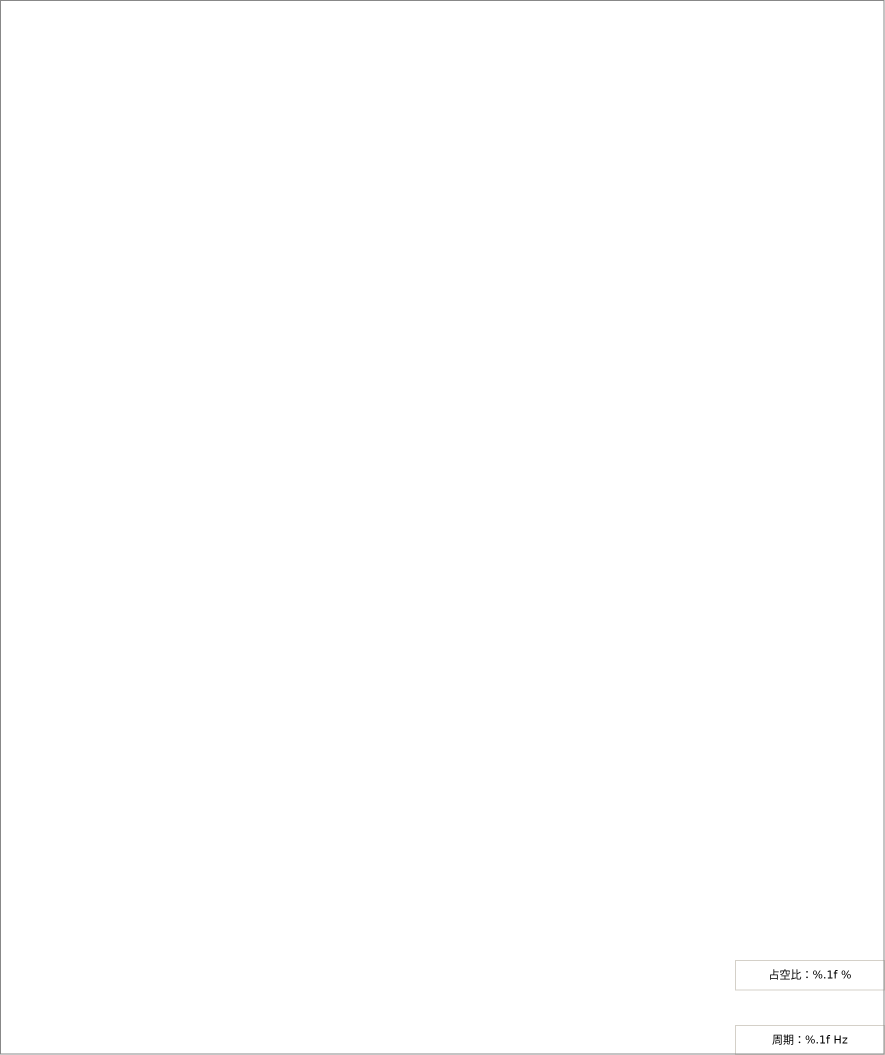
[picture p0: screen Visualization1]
VISUALIZATION Visualization1  // 885x1055
    Textfield (735,960 150x30), "占空比：%.1f %", text variable: MAIN.fDutyCycle
        OnMouseClick: write MAIN.fDutyCycle via Default
    Textfield (735,1025 150x30), "周期：%.1f Hz", text variable: MAIN.fFrequency
        OnMouseClick: write MAIN.fFrequency via Default
END_VISUALIZATION
